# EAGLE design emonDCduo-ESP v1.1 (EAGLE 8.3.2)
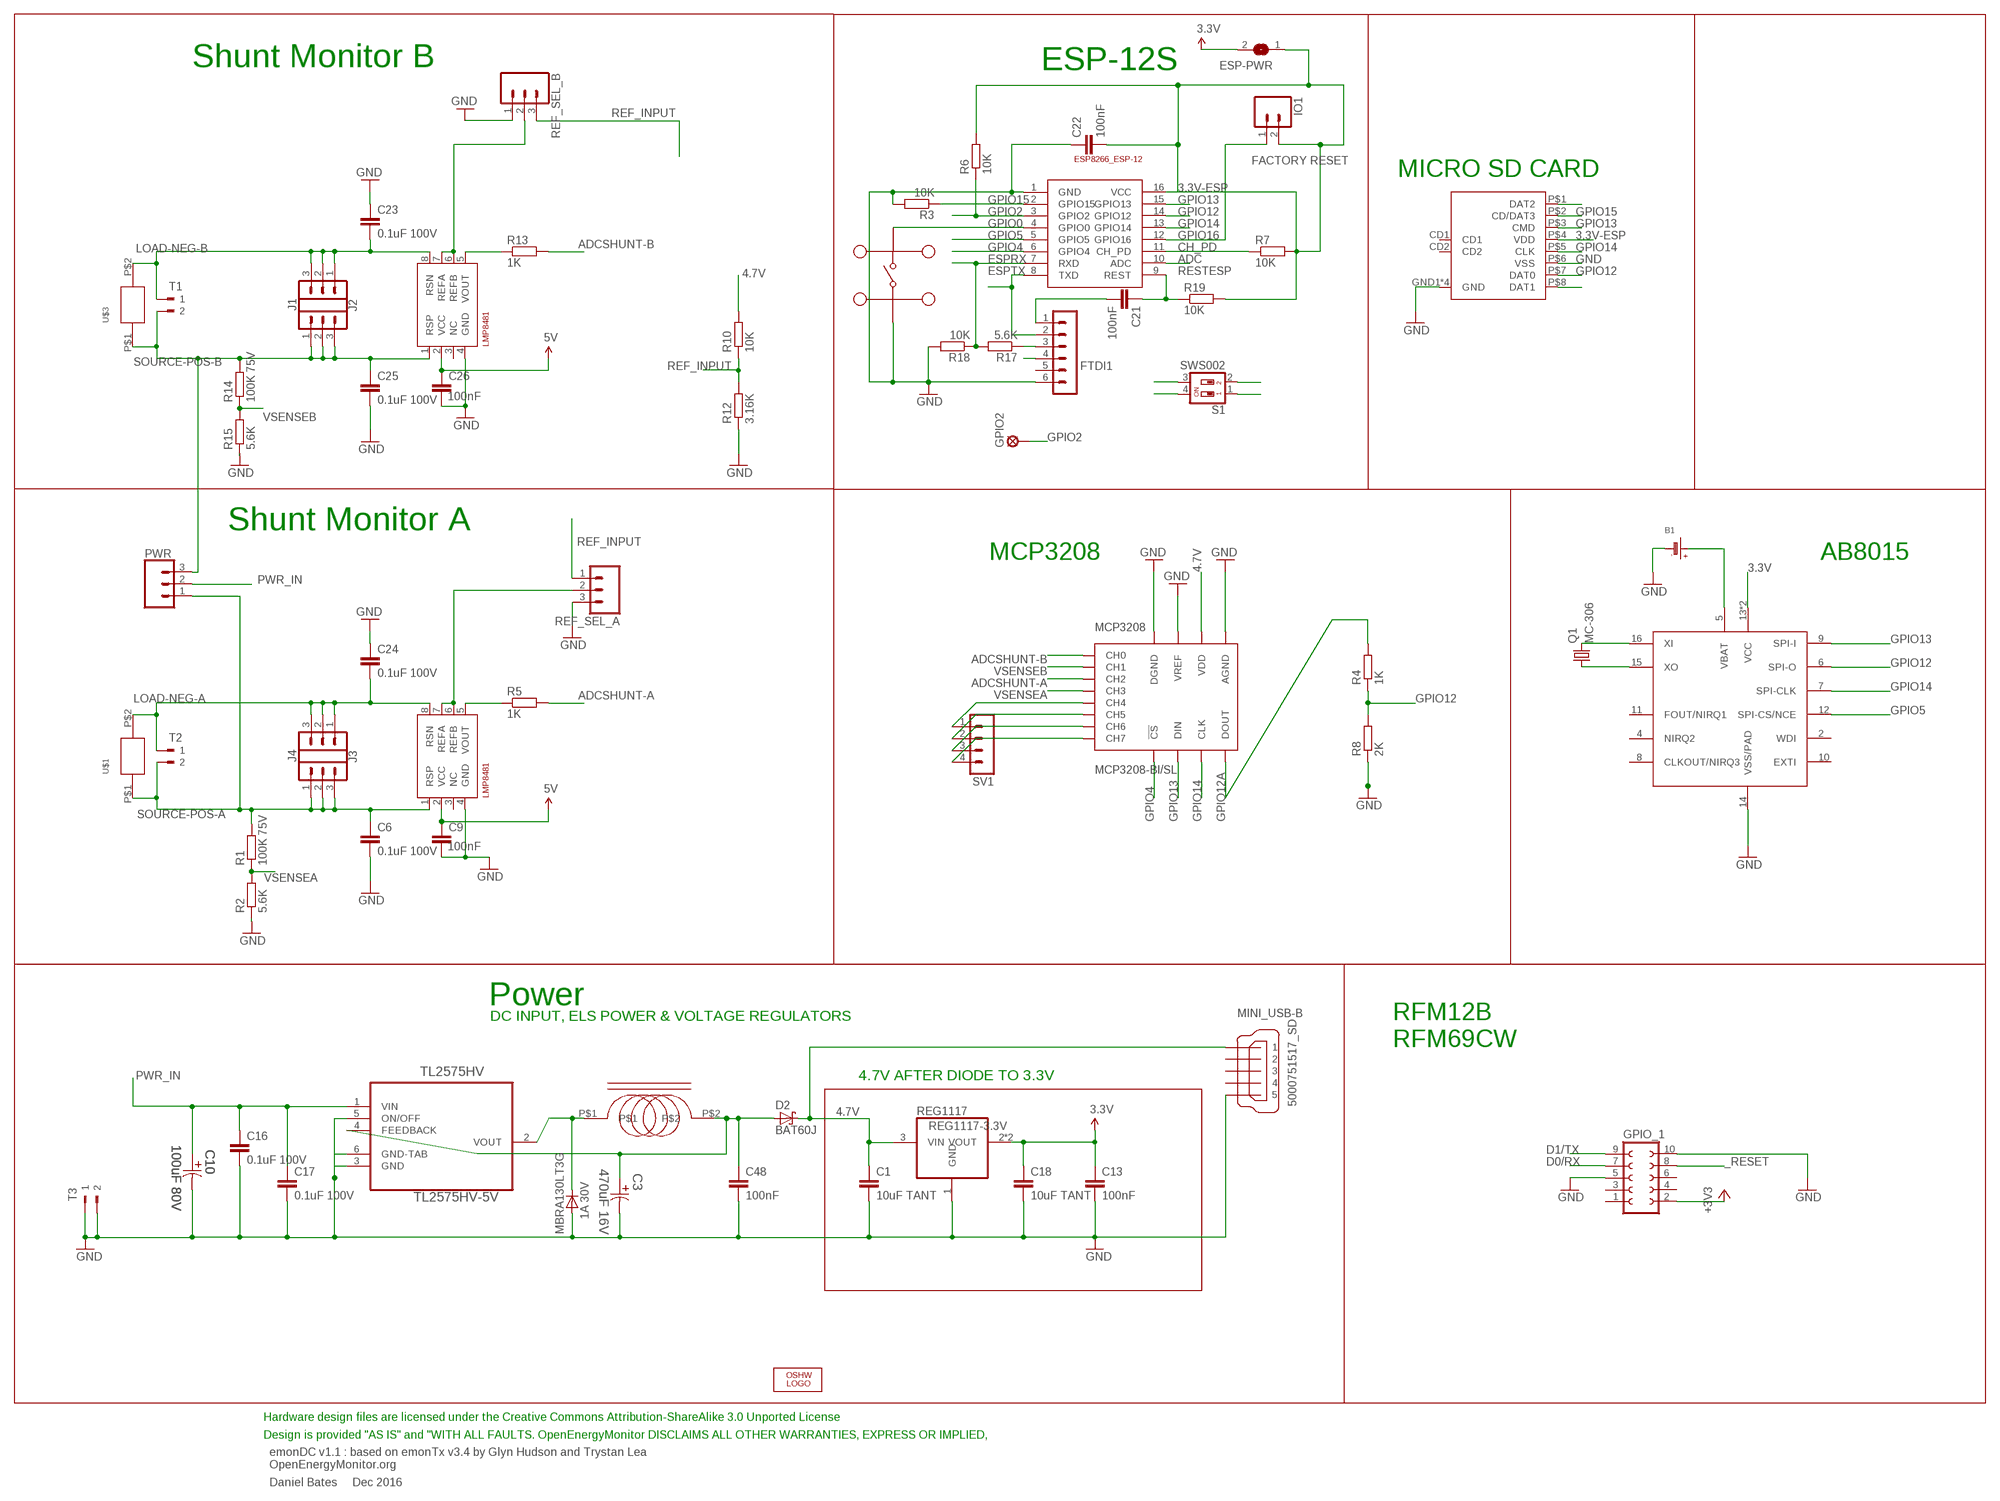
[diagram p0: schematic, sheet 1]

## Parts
AB8015  AB0815_RTC  [QFN16]
B1  BATTERYCR1220_SMT  [CR1220]
C1  10uF TANT  C-EUC0603  [C0603]
C3  470uF 16V  EEE-FK1C471P-CASE-F  [CAPAE830X1050N]
C6  0.1uF 100V  C-EUC0603  [C0603]
C9  100nF  C-EUC0603  [C0603]
C10  100uF 80V  EEV-FK1K101Q-CASE-H13  [CAPAE1350X1400N]
C13  100nF  C-EUC0603  [C0603]
C16  0.1uF 100V  C-EUC0603  [C0603]
C17  0.1uF 100V  C-EUC0603  [C0603]
C18  10uF TANT  C-EUC0603  [C0603]
C21  100nF  C-EUC0603  [C0603]
C22  100nF  C-EUC0603  [C0603]
C23  0.1uF 100V  C-EUC0603  [C0603]
C24  0.1uF 100V  C-EUC0603  [C0603]
C25  0.1uF 100V  C-EUC0603  [C0603]
C26  100nF  C-EUC0603  [C0603]
C48  100nF  C-EUC0603  [C0603]
D1  MBRA130LT3G  [DO-214]
D2  BAT60J  [SOD323_ST]
ESP-12  ESP8266_ESP-12  [ESP8266-ESP12]
ESP-PWR  SJ  [SJ]
FTDI1  FTDI-ESP  MA06-1  [MA06-1]
GPIO2  LSP11  [LSP11]
GPIO_1  FE05-2  [FE05-2]
I1  330uH  SRR0603-331KL  [SRR0603-331KL]
IO1  M02PTH  [1X02]
J1  CONN_03  [1X03]
J2  CONN_03  [1X03]
J3  CONN_03  [1X03]
J4  CONN_03  [1X03]
LOGO1  OSHW_LOGO_6MILX0200-NT  [OSHW_6X200_NOTEXT]
MC2  MC32882  [SWITCH_TACT_MULTICOMP]
MCP3208  MCP3208-BI/SL  [SOIC16]
MINI_USB-B  5000751517_SD  [5000751517_SD]
PWR  CONN_03  [1X03]
Q1  MC-306  [MC-306]
R1  100K 75V  R-EU_R0603  [R0603]
R2  5.6K  R-EU_R0603  [R0603]
R3  10K  R-EU_R0603  [R0603]
R4  1K  R-EU_R0603  [R0603]
R5  1K  R-EU_R0603  [R0603]
R6  10K  R-EU_R0603  [R0603]
R7  10K  R-EU_R0603  [R0603]
R8  2K  R-EU_R0603  [R0603]
R10  10K  R-EU_R0603  [R0603]
R12  3.16K  R-EU_R0603  [R0603]
R13  1K  R-EU_R0603  [R0603]
R14  100K 75V  R-EU_R0603  [R0603]
R15  5.6K  R-EU_R0603  [R0603]
R17  5.6K  R-EU_R0603  [R0603]
R18  10K  R-EU_R0603  [R0603]
R19  10K  R-EU_R0603  [R0603]
REF_SEL_A  2212S-02SG-85  CONN_03  [1X03]
REF_SEL_B  2212S-02SG-85  CONN_03  [1X03]
REG1117  REG1117-3.3V  REG1117-VOUT4  [SOT223]
S1  SWS002  [SMS-002]
SHUNTMON-A  LMP8481  LMP8481-H  [S-PDSO-G08]
SHUNTMON-B  LMP8481  LMP8481-H  [S-PDSO-G08]
SV1  MA04-1  [MA04-1]
T1  180-2  [180-2]
T2  180-2  [180-2]
T3  180-2  [180-2]
TL2575HV  TL2575HV-5V  TL2575HV-05IKTTR  [TO-263]
U$1  EBW_SERIES_10.5MM  [EBW_SERIES_10.5MM]
U$2  MOLEX_MICRO_SD_1040310811  [MOLEX_MICROSD_EXPOSED]
U$3  EBW_SERIES_10.5MM  [EBW_SERIES_10.5MM]

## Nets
3.3V: AB8015.13(VCC) AB8015.PAD(VCC) C13.1 C18.1 ESP-PWR.2 GPIO_1.2 REG1117.2(VOUT) REG1117.4(VOUT) ; supply symbol labelled +3V3
3.3V-ESP: C22.2 ESP-12.16(VCC) ESP-PWR.1 IO1.2 R6.2 R7.2 R19.2 U$2.P$4(VDD)
4.7V [power]: C1.1 C9.1 C26.1 D2.C FTDI1.4 MCP3208.16(VDD) MINI_USB-B.VBUS R10.2 REG1117.3(VIN) SHUNTMON-A.2(VCC) SHUNTMON-B.2(VCC) ; supply symbol labelled 5V
5.0V [power]: C3.1 C48.1 D2.A I1.P$2 TL2575HV.4(FEEDBACK)
_RESET: GPIO_1.8
ADC: ESP-12.10(ADC)
ADCSHUNT-A: MCP3208.3(CH2) R5.2
ADCSHUNT-B: MCP3208.1(CH0) R13.2
CH_PD: ESP-12.11(CH_PD) R7.1
D0/RX: GPIO_1.7 S1.2
D1/TX: GPIO_1.9 S1.1
ESPRX: ESP-12.7(RXD) R17.2 R18.1 S1.4
ESPTX: ESP-12.8(TXD) FTDI1.2 S1.3
GND [thin_power]: AB8015.14(VSS/PAD) B1.- C1.2 C3.2 C6.2 C9.2 C10.2 C13.2 C16.2 C17.2 C18.2 C22.1 C23.1 C24.1 C25.2 C26.2 C48.2 D1.P$2(A) ESP-12.1(GND) FTDI1.6 GPIO_1.5 GPIO_1.10 MC2.P$1 MC2.P$2 MCP3208.9(DGND) MCP3208.14(AGND) MCP3208.15(VREF) MINI_USB-B.GND1 MINI_USB-B.GND2 MINI_USB-B.GND3 R2.1 R3.2 R8.1 R12.1 R15.1 R18.2 REF_SEL_A.3 REF_SEL_B.1 REG1117.1(GND) SHUNTMON-A.4(GND) SHUNTMON-B.4(GND) T3.1 T3.2 TL2575HV.3(GND) TL2575HV.5(ON/OFF) TL2575HV.6(GND-TAB) U$2.GND1(GND) U$2.GND2(GND) U$2.GND3(GND) U$2.GND4(GND) U$2.P$6(VSS)
GPIO0: ESP-12.4(GPIO0) MC2.P$3 MC2.P$4
GPIO2: ESP-12.3(GPIO2) GPIO2.MP R6.1
GPIO4: ESP-12.6(GPIO4) MCP3208.10(!CS)
GPIO5: AB8015.12(SPI-CS/NCE) ESP-12.5(GPIO5)
GPIO12: AB8015.6(SPI-O) ESP-12.14(GPIO12) R4.1 R8.2 U$2.P$7(DAT0)
GPIO12A: MCP3208.12(DOUT) R4.2
GPIO13: AB8015.9(SPI-I) ESP-12.15(GPIO13) MCP3208.11(DIN) U$2.P$3(CMD)
GPIO14: AB8015.7(SPI-CLK) ESP-12.13(GPIO14) MCP3208.13(CLK) U$2.P$5(CLK)
GPIO15 [thin_power]: ESP-12.2(GPIO15) R3.1 U$2.P$2(CD/DAT3)
GPIO16: ESP-12.12(GPIO16) IO1.1
IND: D1.P$1(C) I1.P$1 TL2575HV.2(VOUT)
LOAD-NEG-A: C24.2 J4.1 J4.2 J4.3 SHUNTMON-B.8(RSN) T2.1 U$1.P$2
LOAD-NEG-B: C23.2 J1.1 J1.2 J1.3 SHUNTMON-A.8(RSN) T1.1 U$3.P$2
N$1: MCP3208.5(CH4) SV1.1
N$3: MCP3208.6(CH5) SV1.2
N$4: R13.1 SHUNTMON-A.5(VOUT)
N$5: MCP3208.7(CH6) SV1.3
N$6: R5.1 SHUNTMON-B.5(VOUT)
N$7: U$2.P$1(DAT2)
N$9: MCP3208.8(CH7) SV1.4
N$20: AB8015.5(VBAT) B1.+$1(+)
N$22: AB8015.16(XI) Q1.4
N$23: AB8015.15(XO) Q1.1
N$30: C21.2 FTDI1.1
N$32: U$2.P$8(DAT1)
N$36: FTDI1.3 R17.1
PWR_IN: C10.1 C16.1 C17.1 PWR.2 TL2575HV.1(VIN)
REF_A_INPUT [thin_power]: REF_SEL_A.2 SHUNTMON-B.6(REFB) SHUNTMON-B.7(REFA)
REF_B_INPUT: REF_SEL_B.2 SHUNTMON-A.6(REFB) SHUNTMON-A.7(REFA)
REF_INPUT: R10.1 R12.2 REF_SEL_A.1 REF_SEL_B.3
RESTESP: C21.1 ESP-12.9(REST) R19.1
SOURCE-POS-A: C6.1 J3.1 J3.2 J3.3 PWR.1 R1.2 SHUNTMON-B.1(RSP) T2.2 U$1.P$1
SOURCE-POS-B: C25.1 J2.1 J2.2 J2.3 PWR.3 R14.2 SHUNTMON-A.1(RSP) T1.2 U$3.P$1
VSENSEA: MCP3208.4(CH3) R1.1 R2.2
VSENSEB: MCP3208.2(CH1) R14.1 R15.2
Unconnected: AB8015.2(WDI) AB8015.4(NIRQ2) AB8015.8(CLKOUT/NIRQ3) AB8015.10(EXTI) AB8015.11(FOUT/NIRQ1) FTDI1.5 GPIO_1.1 GPIO_1.3 GPIO_1.4 GPIO_1.6 MINI_USB-B.D+ MINI_USB-B.D- MINI_USB-B.ID SHUNTMON-A.3(NC) SHUNTMON-B.3(NC) U$2.CD1 U$2.CD2

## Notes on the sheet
- Shunt Monitor B | ESP-12S
- FACTORY RESET
- MICRO SD CARD
- Shunt Monitor A
- MCP3208 | AB8015
- Power
- DC INPUT, ELS POWER & VOLTAGE REGULATORS
- RFM12B
  RFM69CW
- 4.7V AFTER DIODE TO 3.3V
- Hardware design files are licensed under the Creative Commons Attribution-ShareAlike 3.0 Unported License
- Design is provided "AS IS" and "WITH ALL FAULTS. OpenEnergyMonitor DISCLAIMS ALL OTHER WARRANTIES, EXPRESS OR IMPLIED,
- emonDC v1.1 : based on emonTx v3.4 by Glyn Hudson and Trystan Lea
  OpenEnergyMonitor.org
- Daniel Bates     Dec 2016

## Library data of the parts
AB8015 = AB0815 RTC:AB0815_RTC
B1 = microbuilder:BATTERY: CR1220 SMT - Digikey: 3001K-ND
C1 C13 C16-C18 C21 C22 C48 = rcl:C-EU: CAPACITOR, European symbol
C3 = Panasonic-EEEFK_EEEFP:EEE-: Aluminum Electrolytic Capacitors,Surface Mount Type; MPN: EEE-FK1C471P; OC_FARNELL: 9695710; OC_NEWARK: 96K9385; PACKAGE: CASE-F; SUPPLIER: PANASONIC; TOLERANCE: ±20 %; VALUE: 470UF; VOLTAGERATING: 16V
C6 C9 C23-C26 = rcl:C-EU: CAPACITOR, European symbol; MPN: C1608X7S2A104K080AB
C10 = Panasonic-EEE-EEV-EEF-ECQ:EEV-: Aluminum Electrolytic Capacitors,Surface Mount Type; MPN: EEVFK1K101Q; OC_FARNELL: 9696113; OC_NEWARK: 96K9484; SUPPLIER: PANASONIC; TOLERANCE: ±20 %; VALUE: 100UF; VOLTAGERATING: 80V
D1 = CASE 403D Diode:MBRA130LT3G: Fast switching diode; MF: ON SEMICONDUCTOR; MPN: MBRA130LT3G; OC_FARNELL: 9555978
D2 = diode:BAT60J: Schottky barrier diode
ESP-12 = ESP8266-ESP12:ESP8266_ESP-12
ESP-PWR = jumper:SJ: SMD solder JUMPER
FTDI1 = JeeLabs:MA06-1: PIN HEADER
GPIO2 = solpad:LSP11: SOLDER PAD
GPIO_1 = con-lsta:FE05-2: FEMALE HEADER; OC_FARNELL: unknown; OC_NEWARK: unknown
I1 = SRR0603-331KL:SRR0603-331KL: SRR0603-331KL; INDUCTANCE: 330uH; MF: BOURNS; MPN: SRR0603-331KL; OC_FARNELL: 2333890
IO1 = SparkFun:M02: Header 2
J1-J4 PWR = SparkFun-Connectors:CONN_03: Multi connection point. Often used as Generic Header-pin footprint for 0.1 inch spaced/style header connections On any of the 0.1 inch spaced packages, you can populate with these: Break Away Headers - Straight (PRT-00116) Break Away Male Headers - Right Angle (PRT-00553) Female Headers (PRT-00115)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
LOGO1 = ohw-logo:OSHW_LOGO_6MIL; OC_FARNELL: unknown
MC2 = multicomp tact switch:MC32882
MCP3208 = MCP3208:MCP3208
MINI_USB-B = 5000751517_sd:5000751517_SD
Q1 = crystal:MC-306: kHz RANGE CRYSTAL UNIT SMD; MPN: MC-306 60.0KHZ 100PPM ,12.5PF; OC_FARNELL: 1278040; OC_NEWARK: 31M5576
R1 R14 = rcl:R-EU_: RESISTOR, European symbol; MPN: MCWR06X1003FTL
R2 R4 R8 R15 = rcl:R-EU_: RESISTOR, European symbol; MPN: MCWR06X5901FTL
R3 R5-R7 R10 R12 R13 R17-R19 = rcl:R-EU_: RESISTOR, European symbol
REF_SEL_A REF_SEL_B = SparkFun-Connectors:CONN_03: Multi connection point. Often used as Generic Header-pin footprint for 0.1 inch spaced/style header connections On any of the 0.1 inch spaced packages, you can populate with these: Break Away Headers - Straight (PRT-00116) Break Away Male Headers - Right Angle (PRT-00553) Female Headers (PRT-00115)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; MF: MULTICOMP; MPN: 2212S-02SG-85; OC_FARNELL: 1593458
REG1117 = burr-brown:REG1117-VOUT4: 800mA and 1A Low Dropout (LDO) Positive Regulator 1.8V, 2.5V, 2.85V, 3.3V, 5V, and Adj; MF: TEXAS INSTRUMENTS; MPN: REG1117; OC_FARNELL: 1097566; OC_NEWARK: 14P6981
S1 = smd-special:SWS002: SMD Dip Switch 2 pol.
SHUNTMON-A = lmp8481b:LMP8481: LMP8481MM-H/NOPB 100V/V; MF: TEXAS INSTRUMENTS; MPN: LMP8481MME-S/NOPB; OC_FARNELL: 2322044
SHUNTMON-B = lmp8481b:LMP8481: LMP8481MM-H/NOPB 100V/V; MF: TEXAS INSTRUMENTS; MPN: LMP8481MME-H/NOPB; OC_FARNELL: 2322044
SV1 = con-lstb:MA04-1: PIN HEADER; OC_FARNELL: unknown; OC_NEWARK: unknown
T1-T3 = con-weidmueller-sl35:180-2: WEIDMUELLER CLAMP CONNECTOR; OC_FARNELL: unknown; OC_NEWARK: unknown
TL2575HV = TL2575HV:TL2575HV; MF: TEXAS INSTRUMENTS; MPN: LM2575HVS-15/NOPB; OC_FARNELL: 2492609
U$1 U$3 = EBW series shunt:EBW_SERIES_10.5MM
U$2 = MOLEX MICRO SD [exposed pins]:MOLEX_MICRO_SD_1040310811

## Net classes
2 thin_power: width 0.254 mm

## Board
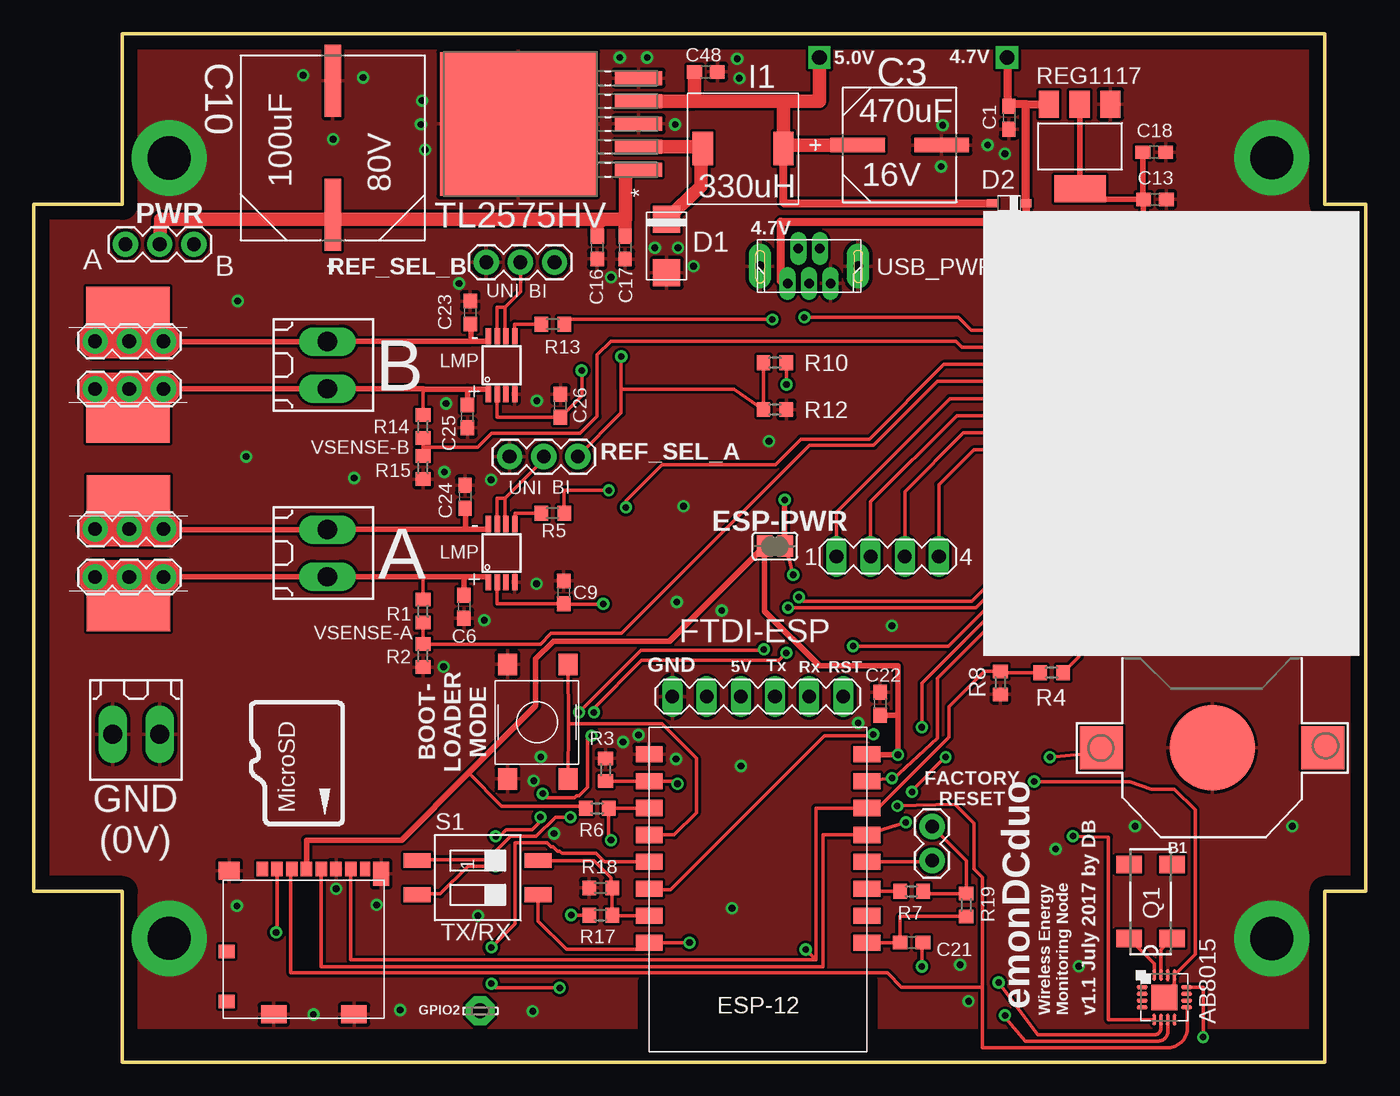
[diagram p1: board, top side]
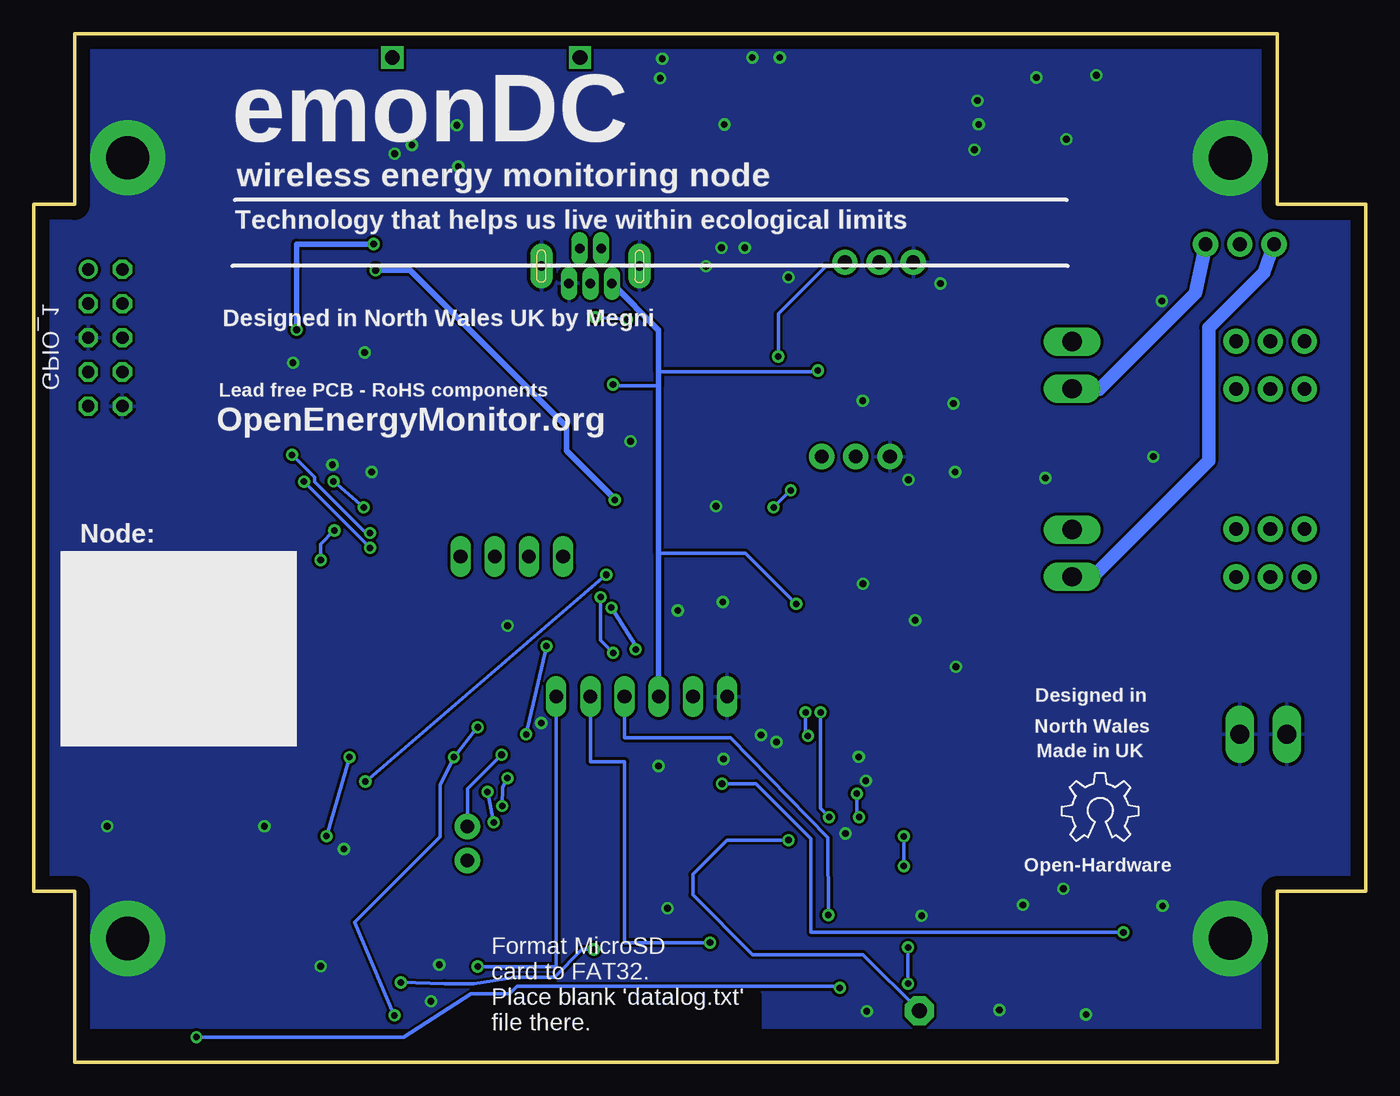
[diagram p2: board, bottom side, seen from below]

Size 99.06 x 76.45 mm. Coordinates in mm from the lower left corner, seen from the top.
Outline: 6.6,63.75 6.6,76.45 96.01,76.45 96.01,63.75 99.06,63.75 99.06,12.7 96.01,12.7 96.01,0 6.6,0 6.6,12.7 0,12.7 0,63.75 6.6,63.75
Copper layers (1*16): Top 0.035mm / dielectric 1.5mm / Bottom 0.035mm
Design rules "default *": minimum track width 10mil, minimum drill 19mil, track to track 8mil, track to pad 8mil, pad to pad 8mil, via to via 8mil, smd to smd 8mil, copper to edge 40mil, drill to drill 8mil, minimum pad ring 10mil, minimum via ring 8mil, stop-mask expansion 4mil, vias tented up to drill 0mil, thermal gap 10mil
tRestrict: area 45.2,2.3 to 62.5,6.1
bRestrict: area 45.2,2.3 to 62.5,5.1

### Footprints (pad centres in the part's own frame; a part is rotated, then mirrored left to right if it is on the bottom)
QFN16 = smd 0.85 x 0.3: 1 -1.655,0.75; 2 -1.655,0.25; 3 -1.655,-0.25; 4 -1.655,-0.75; 9 1.655,-0.75; 10 1.655,-0.25; 11 1.655,0.25; 12 1.655,0.75 | smd 0.3 x 0.85: 5 -0.75,-1.655; 6 -0.25,-1.655; 7 0.25,-1.655; 8 0.75,-1.655; 13 0.75,1.655; 14 0.25,1.655; 15 -0.25,1.655; 16 -0.75,1.655 | smd 1.9 x 1.9: PAD 0,0
CR1220 = smd 3.2 x 3.2: +$1 -8.225,0; +$2 8.225,0 | smd 6.35 x 6.35: - 0,0
C0603 = smd 1.1 x 1: 1 -0.85,0; 2 0.85,0
CAPAE830X1050N = smd 4.064 x 1.092: 1 -3.124,0; 2 3.124,0
CAPAE1350X1400N = smd 5.359 x 1.194: 1 -4.978,0; 2 4.978,0
DO-214 = smd 2 x 2: P$1 -2,0; P$2 2,0
SOD323_ST = smd 0.8 x 0.6: A 1.25,0; C -1.25,0
ESP8266-ESP12 = smd 2 x 1.2: 1 16.2,2; 2 16.2,4; 3 16.2,6; 4 16.2,8; 5 16.2,10; 6 16.2,12; 7 16.2,14; 8 16.2,16; 9 0,16; 10 0,14; 11 0,12; 12 0,10; 13 0,8; 14 0,6; 15 0,4; 16 0,2
SJ = smd 1.168 x 1.6: 1 -0.762,0; 2 0.762,0
MA06-1 = drill 1.016 long: 1 0,0; 2 2.54,0; 3 5.08,0; 4 7.62,0; 5 10.16,0; 6 12.7,0
LSP11 = drill 1.118 pad 2.159 octagon: MP 0,0
FE05-2 = drill 0.914: 1 -5.08,1.27 | drill 0.914 octagon: 2 -5.08,-1.27; 3 -2.54,1.27; 4 -2.54,-1.27; 5 0,1.27; 6 0,-1.27; 7 2.54,1.27; 8 2.54,-1.27; 9 5.08,1.27; 10 5.08,-1.27
SRR0603-331KL = smd 1.5 x 2.5: P$1 -3,0; P$2 3,0
1X02 = drill 1.016 pad 1.88: 1 0,0; 2 2.54,0
1X03 = drill 1.016 pad 1.88: 1 0,0; 2 2.54,0; 3 5.08,0
SWITCH_TACT_MULTICOMP = smd 1.6 x 1.4: P$1 -1.1,5.3; P$2 7.4,5.3; P$3 -1.1,0.8; P$4 7.4,0.8
SOIC16 = smd 0.635 x 1.524: 1 -4.445,-2.695; 2 -3.175,-2.695; 3 -1.905,-2.695; 4 -0.635,-2.695; 5 0.635,-2.695; 6 1.905,-2.695; 7 3.175,-2.695; 8 4.445,-2.695; 9 4.445,2.695; 10 3.175,2.695; 11 1.905,2.695; 12 0.635,2.695; 13 -0.635,2.695; 14 -1.905,2.695; 15 -3.175,2.695; 16 -4.445,2.695
5000751517_SD = drill 0.7 pad 1.016 long: D+ 0,-1.3; D- -0.8,1.3; GND1 1.6,-1.3; ID 0.8,1.3; VBUS -1.6,-1.3 | drill 0.7 pad 1.676 long: GND2 3.65,0; GND3 -3.65,0
MC-306 = smd 1.3 x 1.9: 1 -2.75,-1.6; 2 2.75,-1.6; 3 2.75,1.6; 4 -2.75,1.6
R0603 = smd 1 x 1.1: 1 -0.85,0; 2 0.85,0
SOT223 = smd 1.499 x 2.007: 1 -2.261,-3.15; 2 0.025,-3.15; 3 2.311,-3.15 | smd 3.81 x 2.007: 4 0,3.15
SMS-002 = smd 1.092 x 2.007: 1 -1.27,-4.496; 2 1.27,-4.496; 3 1.27,4.496; 4 -1.27,4.496
S-PDSO-G08 = smd 0.4 x 1.2: 1 -0.975,-2.157; 2 -0.325,-2.157; 3 0.325,-2.157; 4 0.975,-2.157; 5 0.975,2.157; 6 0.325,2.157; 7 -0.325,2.157; 8 -0.975,2.157
MA04-1 = drill 1.016 long: 1 -3.81,0; 2 -1.27,0; 3 1.27,0; 4 3.81,0
180-2 = drill 1.422 long: 1 -1.75,0; 2 1.75,0
TO-263 = smd 1.041 x 3.505: 1 -3.404,-8.788; 2 -1.702,-8.788; 3 0,-8.788; 4 1.702,-8.788; 5 3.404,-8.788 | smd 10.668 x 11.659: 6 0,0.152
EBW_SERIES_10.5MM = smd 3 x 6.2: P$1 -4.3,0; P$2 4.3,0
MOLEX_MICROSD_EXPOSED = smd 1.195 x 1.005: CD1 5.349,0.435; CD2 5.349,4.135 | smd 1.907 x 1.348: GND1 -4.112,5.104; GND2 1.853,5.104 | smd 1.17 x 1.793: GND3 -6.134,-5.352 | smd 1.551 x 1.348: GND4 5.167,-5.577 | smd 0.851 x 1.092: P$1 2.707,-5.703; P$2 1.617,-5.703; P$3 0.522,-5.699; P$4 -0.586,-5.701; P$5 -1.676,-5.703; P$6 -2.769,-5.703; P$7 -3.875,-5.701 | smd 0.749 x 1.092: P$8 -4.935,-5.701

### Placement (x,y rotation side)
AB8015  84.07,4.83 0 top
B1  87.63,23.37 0 top
C1  72.52,70.21 270 top
C3  64.39,68.17 0 top
C6  32,33.86 270 top
C9  39.42,34.93 90 top
C10  22.25,67.96 90 top
C13  83.38,64.13 0 top
C16  41.9,60.55 270 top
C17  43.97,60.55 270 top
C18  83.32,67.64 0 top
C21  65.28,8.89 0 top
C22  62.94,26.64 270 top
C23  32.46,55.73 270 top
C24  32.08,42.04 270 top
C25  32.26,48.01 270 top
C26  39.17,48.8 90 top
C48  49.99,73.61 0 top
D1  47.06,60.67 270 top
D2  72.53,63.85 180 top
ESP-12  61.98,24.89 180 top
ESP-PWR  55.12,38.35 0 top
FTDI1  60.2,27.18 180 top
GPIO2  33.21,3.81 0 top
GPIO_1  93.73,53.85 270 top
I1  52.76,67.91 0 top
IO1  66.8,14.99 90 top
J1  4.57,53.59 0 top
J2  4.57,50.04 0 top
J3  4.57,36.07 0 top
J4  4.57,39.62 0 top
LOGO1  22.6,16.43 0 bottom
MC2  40.53,22.17 90 top
MCP3208  74.54,49.96 270 top
MINI_USB-B  57.66,59.18 0 top
PWR  6.84,60.8 0 top
Q1  83.06,11.94 90 top
R1  28.96,33.53 90 top
R2  28.96,30.23 90 top
R3  42.53,21.74 90 top
R4  75.69,28.96 0 top
R5  38.6,40.81 0 top
R6  41.91,18.87 180 top
R7  65.28,12.7 0 top
R8  71.88,28.19 90 top
R10  55.12,52 0 top
R12  55.12,48.51 180 top
R13  38.61,54.86 0 top
R14  28.96,47.24 90 top
R15  28.96,44.2 90 top
R17  42.16,10.92 0 top
R18  42.16,12.95 180 top
R19  69.34,11.68 90 top
REF_SEL_A  40.47,45.01 180 top
REF_SEL_B  33.65,59.46 0 top
REG1117  77.8,68.07 180 top
S1  33.02,13.72 270 top
SHUNTMON-A  34.8,51.82 0 top
SHUNTMON-B  34.8,37.85 0 top
SV1  63.5,37.59 0 top
T1  21.84,51.82 270 top
T2  21.84,37.85 270 top
T3  7.62,24.38 180 top
TL2575HV  36.19,69.74 90 top
U$1  7.05,37.82 90 top
U$2  19.71,8.66 180 top
U$3  7.02,51.83 90 top

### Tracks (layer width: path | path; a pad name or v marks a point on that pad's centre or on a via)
3.3V  (via drill 0.5)
  Top 0.254: AB8015.13 84.84,5.84 84.52,5.53 84.52,4.89 84.2,4.89 AB8015.PAD | 55.94,38.39 ESP-PWR.2 55.94,38.23 56.45,36.29 | 92.46,58.86 GPIO_1.2 | v74.39,20.86 81.5,20.86 83.09,20.29 84.84,20.29 86.36,18.76 86.36,8.02 AB8015.13 | 56.52,36.32 56.61,36.23 | 84.84,6.64 AB8015.13
  Top 0.406: REG1117.2 77.76,71.22 | 82.51,58.86 92.46,58.86 | 82.51,58.86 v73.63,58.86 | REG1117.4 78.6,64.13 C13.1 | C13.1 82.47,64.18 C18.1 | C13.1 82.51,64.11 82.51,58.86 | v55.84,41.8 55.84,38.49 55.94,38.39 | 56.45,36.29 56.48,36.26 v56.48,36.23 56.48,36.29 56.52,36.32
  Bottom 0.254: v56.48,36.23 v74.39,20.86
  Bottom 0.406: v73.63,58.86 71.06,58.86 59.44,47.24 59.44,45.45 55.87,41.89 55.87,41.83 v55.84,41.8
3.3V-ESP  (via drill 0.5)
  Top 0.254: R7.2 66.13,12.53 R19.2 69.34,14.99 IO1.2 | R6.2 40.89,19.04 34.81,19.04 32.35,21.5
  Top 0.406: 64.26,25.91 64.26,29.46 58.42,29.46 54.36,33.53 ESP-PWR.1 47.29,31.28 38.65,31.28 37.34,29.97 37.34,26.49 32.35,21.5 27.35,16.51 20.3,16.51 U$2.P$4 | 64.26,25.91 v64.26,22.86 62.01,22.86 ESP-12.16 | C22.2 64.15,25.8 64.26,25.91
  Bottom 0.254: v64.26,22.86 66.8,20.32 IO1.2
4.7V  (via drill 0.5, 1.1)
  Top 0.254: SHUNTMON-A.2 34.47,47.95 C26.1 40.76,49.54 40.76,51.36 40.75,51.36 v40.75,51.41 | SHUNTMON-B.2 34.47,34.08 C9.1 39.46,34.04 42.42,34.04 42.39,34.07 v42.36,34.07 | R10.2 55.98,51.98 v55.98,50.38
  Top 0.406: D2.C 73.96,63.85 | 72.39,71.06 C1.1 72.52,71.22 | 73.78,62.48 73.79,62.48 v73.79,60.81 | v79.5,54.44 77.27,54.44 MCP3208.16 | MINI_USB-B.VBUS 55.86,58.08 55.56,58.08
  Top 0.61: v72.39,74.68 72.39,71.06 | 73.78,71.22 D2.C 73.78,62.48 55.56,62.48 55.56,58.08 | 73.78,71.22 REG1117.3 | 73.78,71.22 72.52,71.22
  Bottom 0.254: v55.98,50.38 55.9,50.29 52.58,50.29 | v40.75,51.41 40.85,51.31 52.58,51.31 | v42.36,34.07 46.14,37.85 52.58,37.85
  Bottom 0.406: v79.5,54.44 79.5,60.81 v73.79,60.81 | FTDI1.4 52.58,37.85 52.58,50.29 52.58,51.31 52.58,54.4 MINI_USB-B.VBUS
5.0V  (via drill 1.1)
  Top 0.61: D2.A 55.76,63.85 I1.P$2
  Top 1.016: TL2575HV.4 49.14,71.44 | 49.14,71.44 C48.1 | 55.76,71.44 I1.P$2 55.5,68.17 C3.1 | 55.76,71.44 49.14,71.44 | v58.42,74.68 58.42,71.44 55.76,71.44
ADCSHUNT-A  (via drill 0.48)
  Top 0.254: v42.77,42.51 39.43,42.51 39.43,40.93 R5.2 | v44.04,41.24 44.04,41.72 46.74,44.42 55.15,44.42 57.05,46.32 62.14,46.32 67.69,51.88 71.82,51.88 MCP3208.3
  Bottom 0.254: v44.04,41.24 v42.77,42.51
ADCSHUNT-B  (via drill 0.48)
  Top 0.254: v57.31,55.37 68.77,55.37 69.72,54.42 71.82,54.42 MCP3208.1 | R13.2 39.43,54.9 39.43,55.21 54.99,55.21 v54.92,55.21
  Bottom 0.254: v54.92,55.21 v57.31,55.37
CH_PD
  Top 0.254: ESP-12.11 61.98,12.7 R7.1
D0/RX  (via drill 0.48)
  Top 0.254: v34.35,14.57 32.29,14.57 30.23,12.51 28.64,12.51 S1.2 | v34.35,16.8 34.67,16.8 35.15,17.27 37.05,17.27 37.69,17.91 v37.69,18.23 | v37.85,19.97 38.16,19.65 40.23,19.65 40.39,19.81 40.55,19.81 41.18,20.45 41.18,24.26 v41.5,24.26 | v41.66,26 41.66,26.32 45.21,29.88 55.42,29.88 v55.97,30.43 55.96,30.22 | v56.9,34.58 57.21,34.26 69.75,34.26 73.25,37.75 73.25,39.34 v74.04,39.34 | v79.85,45.15 79.66,44.89 82.52,47.75 89.92,47.75 92.2,50.04 93.22,50.04 94.23,51.05 94.8,51.05 95,51.25 GPIO_1.7
  Bottom 0.254: v34.35,16.8 v34.35,14.57 | v37.69,18.23 37.85,18.38 v37.85,19.97 | v41.5,24.26 41.66,24.42 v41.66,26 | v74.04,39.34 74.36,39.34 78.17,43.15 78.17,43.47 v79.85,45.15 | v55.97,30.43 56.9,31.35 v56.9,34.58
D1/TX  (via drill 0.48)
  Top 0.254: v39.91,18.23 38.8,18.23 37.37,16.8 35.47,16.8 33.72,15.05 28.64,15.05 S1.1 | v40.55,26 45.15,30.61 54.22,30.61 v54.29,30.68 | v56.1,33.78 70.07,33.78 74.04,37.75 v74.04,38.23 | v78.96,43.15 82.3,46.48 93.98,46.48 95,47.5 GPIO_1.9 95,48.7
  Bottom 0.254: v39.91,18.23 40.55,18.86 v40.55,26 | v54.29,30.68 54.32,31.02 v56.1,33.78 | v78.96,43.15 v74.04,38.23
ESPRX
  Top 0.254: ESP-12.7 42.79,10.89 R17.2 R18.1 42.93,13.04 42.93,13.72 41.66,14.99 S1.4
ESPTX  (via drill 0.5)
  Top 0.254: v48.77,8.89 ESP-12.8 45.27,8.38 39.62,8.38 37.52,10.49 S1.3
  Bottom 0.254: v48.77,8.89 55.12,8.89 55.12,22.35 57.66,22.35 FTDI1.2
GND  (via drill 0.5, 3.2 pad 5.59)
  Top 0.254: ESP-12.1 46.06,22.61
  Top 0.406: U$2.GND2 | U$2.P$6 22.48,14.39 | 25.86,13.97 25.91,13.97 25.96,14.02
  other vias: 10.08,67.21 92.07,67.23 52.47,73.15 10.08,9.2 92.07,9.2 33.51,32.85 15.17,56.58 30.55,43.87 37.41,49.17 70.94,68.18 30.66,48.96 37.39,35.57 47.77,22.53 51.93,11.44 22.49,12.89 42.93,58.34 49.07,59.16 67.59,69.65 47.7,69.7 28.88,71.47 20.04,73.36 24.49,73.2 15.81,45.01 30.48,29.4 34.01,43.3 20.81,3.54 47.92,60.54 44.98,24.32 25.51,11.7 61.31,25.22 15.12,11.62 38.69,17 31.64,57.88 23.83,43.43 43.83,23.8 37.18,20.93 37.71,22.7 33.04,10.88 27.25,3.88 37.11,3.79 46.19,60.53 67.48,66.58 72.22,67.52 52.32,74.58 29.11,67.83 28.79,69.71 43.59,74.69 45.62,74.69 22.27,68.6 68.89,7.24 77.71,7.13 75.99,15.85 93.58,17.54 81.9,17.54 48.33,41.33 47.82,34.21 51.17,33.58 63.82,32.44 69.52,4.54 52.6,22.02 73.93,43.87 79.77,52 74.44,52.76 76.85,44.42 54.68,46.15
  pour Bottom (isolate 0.127): 6.86,76.2 6.86,63.5 0.25,63.5 0.25,12.95 6.86,12.95 6.86,2.54 95.76,2.54 95.76,12.95 98.81,12.95 98.81,63.5 95.76,63.5 95.76,76.2
  pour Top (isolate 0.127): 6.86,76.2 6.86,63.5 0.25,63.5 0.25,12.95 6.86,12.95 6.86,2.54 95.76,2.54 95.76,12.95 98.81,12.95 98.81,63.5 95.76,63.5 95.76,76.2
GPIO0
  Top 0.254: MC2.P$3 39.77,25.15 | 39.77,25.15 MC2.P$4 | ESP-12.4 47.63,16.89 49.28,18.54 49.28,22.61 46.74,25.15 39.77,25.15
GPIO2  (via drill 0.5)
  Top 0.254: ESP-12.3 42.78,18.89 R6.1 42.76,16.68 v42.93,16.51
  Bottom 0.254: v42.93,16.51 47.5,16.51 50.04,13.97 50.04,12.45 45.6,8.01 37.4,8.01 GPIO2.MP
GPIO4  (via drill 0.48)
  Top 0.254: 45.32,12.89 ESP-12.6 45.78,12.83 47.37,12.83 58.8,24.26 62.14,24.26 v62.44,24.38 | v74.52,41.24 74.83,40.93 74.83,37.75 68.01,30.93 v60.93,30.93 | MCP3208.10 77.38,46.64 77.69,46.64 78.33,46.01 78.33,45 77.66,44.33 77.66,43.91 76.92,43.17 v76.76,43.17
  Bottom 0.254: v74.52,41.24 v76.76,43.17 | v62.44,24.38 v60.93,30.93
GPIO5  (via drill 0.48)
  Top 0.254: v86.95,1.87 86.96,2.76 86.96,5.58 AB8015.12 | v34.04,8.54 35.78,10.29 35.78,16.32 38.16,16.32 38.48,16 38.64,16 38.96,15.68 39.12,15.68 39.28,15.53 41.82,15.53 42.45,14.89 45.62,14.89 ESP-12.5 | v34.04,5.84 34.35,5.53 v39.12,5.53
  Bottom 0.254: v34.04,8.54 v34.04,5.84 | v86.95,1.87 85.63,1.87 71.53,1.87 66.55,5.08 63.68,5.08 63.13,5.63 39.22,5.63 v39.12,5.53
GPIO12  (via drill 0.5)
  Top 0.254: 58.17,7.62 23.59,7.62 U$2.P$7 | 58.17,7.62 58.17,18.89 ESP-12.14 61.98,18.86 62.77,18.86 68.07,24.16 68.07,26.42 70.7,29.04 R8.2 71.97,28.96 R4.1 | AB8015.6 83.82,2.54 arc-90 83.31,2.03 74.68,2.03 v71.75,5.93 | 58.17,7.62 v57.4,8.38
  Bottom 0.254: v71.75,5.93 68.52,5.84 67.24,5.83 66.3,5.83 63.27,6.33 60.34,6.33 58.28,8.38 v57.4,8.38
GPIO12A  (via drill 0.5)
  Top 0.254: 77.22,49.34 MCP3208.12 76.61,48.71 76.34,48.71 75.77,48.14 75.77,40.45 76.69,39.52 v76.7,39.52 | R4.2 77.72,30.14 v77.72,37.33
  Bottom 0.254: v76.7,39.52 77.72,38.5 v77.72,37.34 v77.72,37.33
GPIO13  (via drill 0.48)
  Top 0.254: MCP3208.11 77.38,48.07 78.33,48.07 78.8,47.59 78.8,44.74 78.17,44.1 78.17,39.5 67.21,28.54 67.21,24.1 63.88,21.05 v63.82,21.12 61.98,20.92 ESP-12.15 | U$2.P$3 19.11,14.26 19.11,6.64 63.47,6.64 64.52,5.59 70.55,5.59 | AB8015.9 85.79,3.94 85.79,2.57 arc-90 84.37,1.08 70.56,1.08 70.55,5.59 | v64.23,19.05 68.48,19.18 69.91,17.75 69.91,14.38 70.55,13.75 70.55,5.59
  Bottom 0.254: v63.82,21.12 64.2,20.45 v64.23,19.05
GPIO14  (via drill 0.48, 0.5)
  Top 0.254: U$2.P$5 21.39,7.11 58.67,7.11 58.67,16.89 ESP-12.13 61.98,16.96 62,16.94 v64.85,17.83 | v67.81,22.68 67.8,22.7 65.28,20.13 v65.31,20.09 | MCP3208.13 77.22,50.61 76.1,50.61 75.31,49.82 75.31,37.43 66.05,28.17 66.05,24.92 66.04,24.91 v66.04,24.89 | v72.23,3.48 72.23,3.14 72.39,3.56 72.25,3.3 73.72,1.58 83.62,1.58 arc90 84.33,2.29 AB8015.7 arc90 AB8015.7
  Bottom 0.254: v64.85,17.83 v65.31,20.09 | v72.23,3.48 72.3,3.56 75.18,10.41 68.83,16.76 68.83,20.57 67.84,22.65 v67.81,22.68 66.12,24.82 v66.04,24.89
GPIO15  (via drill 0.5)
  Top 0.254: ESP-12.2 R3.1 47.88,20.89 v47.88,20.7 | v18.03,9.65 18.09,9.65 U$2.P$2
  Bottom 0.254: v47.88,20.7 45.35,20.7 41.25,16.6 41.25,9.65 v18.03,9.65
GPIO16
  Top 0.254: IO1.1 66.71,14.89 ESP-12.12
IND
  Top 1.016: TL2575HV.2 49.63,68.04 | 49.63,68.04 I1.P$1 | 49.63,68.04 49.63,65.1 D1.P$1
LOAD-NEG-A
  Top 0.406: 32.12,39.62 33.82,39.62 SHUNTMON-B.8 | C24.2 32.12,41.19 32.12,39.62 | J4.1 J4.2 J4.3 | 9.68,39.6 T2.1 21.87,39.62 32.12,39.62
  Top 2.54: J4.1 J4.3 9.68,39.6 | J4.2 7.11,42.06 U$1.P$2
LOAD-NEG-B
  Top 0.406: 32.51,53.59 33.82,53.59 SHUNTMON-A.8 | C23.2 32.51,54.88 32.51,53.59 | J1.3 9.68,53.57 T1.1 21.87,53.59 32.51,53.59
  Top 2.54: J1.1 J1.2 | J1.2 J1.3 | U$3.P$2 7.02,53.69 J1.2
N$1
  Top 0.254: MCP3208.5 68.12,49.33 59.69,40.89 SV1.1
N$2
  Top 0.406: 77.72,64.9 77.8,64.9 77.8,71.15
N$3
  Top 0.254: MCP3208.6 68.63,48.06 62.23,41.66 SV1.2
N$4
  Top 0.254: SHUNTMON-A.5 35.77,54.86 R13.1
N$5
  Top 0.254: MCP3208.7 69.14,46.79 64.77,42.42 SV1.3
N$6
  Top 0.254: SHUNTMON-B.5 35.81,40.81 R5.1
N$9
  Top 0.254: MCP3208.8 69.9,45.52 67.31,42.93 SV1.4
N$20  (via drill 0.48)
  Top 0.254: v75.56,22.67 79.79,23.08 80.07,24.1 B1.+$1 | v77.28,16.81 79.91,16.73 79.91,3.14 83.25,3.14 AB8015.5
  Bottom 0.254: v77.28,16.81 v75.56,22.67
N$22
  Top 0.254: Q1.4 83.32,7.32 AB8015.16
N$23
  Top 0.254: Q1.1 83.82,8.35 AB8015.15
N$30  (via drill 0.5)
  Top 0.254: v66.04,7.11 66.04,8.89 C21.2
  Bottom 0.254: FTDI1.1 60.2,7.11 v66.04,7.11
N$36  (via drill 0.5)
  Top 0.254: v39.97,10.94 R17.1
  Bottom 0.254: FTDI1.3 55.12,24.13 47.24,24.13 39.99,16.68 v39.97,10.94
PWR_IN
  Top 1.016: 44.27,66.33 TL2575HV.1 44.01,66.33 44.01,62.66 43.94,62.66 | PWR.2 9.46,62.66 21.93,62.66 | 43.94,62.66 42.29,62.66 41.9,62.27 | C16.1 41.9,62.27 | C17.1 43.97,62.63 43.94,62.66 | 21.93,62.66 C10.1 | 41.9,62.27 41.9,62.66 21.93,62.66
REF_A_INPUT
  Top 0.254: REF_SEL_A.2 37.93,44.79 35.05,41.91 | 35.05,41.91 35.05,40.07 SHUNTMON-B.6 | SHUNTMON-B.7 34.47,41.91 35.05,41.91
REF_B_INPUT
  Top 0.254: 36.2,57.28 35.05,56.13 | 35.05,56.13 35.05,54.04 SHUNTMON-A.6 | REF_SEL_B.2 36.2,57.28 | 36.2,57.28 | SHUNTMON-A.7 34.47,56.13 35.05,56.13
REF_INPUT  (via drill 0.5)
  Top 0.254: 43.69,50.04 v43.69,52.45 | 43.69,50.04 43.69,48.26 40.47,45.04 REF_SEL_A.1 | R10.1 R12.2 52.07,50.04 43.69,50.04
  Bottom 0.254: v43.69,52.45 43.69,55.63 40.13,59.18 39.01,59.18 REF_SEL_B.3
RESTESP
  Top 0.254: ESP-12.9 C21.1 64.43,10.83 R19.1
SOURCE-POS-A
  Top 0.254: R1.2 28.96,36.07
  Top 0.406: 32,36.07 28.96,36.07 28.96,36.1 T2.2 9.68,36.1 | 32,36.07 33.82,36.07 SHUNTMON-B.1 | C6.1 32,36.07 | J3.1 4.83,35.81 5.08,36.07 J3.2 J3.3
  Top 2.54: J3.1 J3.3 9.68,36.1 | J3.2 7.11,33.58 U$1.P$1
  Bottom 1.016: 22.86,36.07 21.87,36.07 T2.2 20.29,36.1 11.68,44.7 11.68,54.61 7.6,58.7 PWR.1
SOURCE-POS-B
  Top 0.254: R14.2 28.96,50.04
  Top 0.406: 32.26,50.04 28.96,50.04 28.96,50.07 T1.2 9.68,50.07 J2.3 J2.2 J2.1 | 32.26,50.04 33.69,50.04 33.82,49.91 SHUNTMON-A.1 | C25.1 32.26,50.04
  Top 2.54: J2.1 J2.3 | J2.2 7.11,47.63 U$3.P$1
  Bottom 1.016: PWR.3 12.68,57.17 19.81,50.04 21.82,50.04 T1.2
VSENSEA
  Top 0.254: R2.2 R1.1 | R2.2 37.69,31.08 38.48,31.88 43.72,31.88 57.69,45.85 62.45,45.85 67.21,50.61 71.82,50.61 MCP3208.4 | R2.2
VSENSEB
  Top 0.254: 28.96,44.96 R15.2 28.96,45.72 | R14.1 28.96,45.72 | MCP3208.2 69.03,53.14 68.58,53.59 42.93,53.59 41.91,52.58 41.91,48.01 40.64,46.74 34.04,46.74 33.02,45.72 28.96,45.72

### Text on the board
tPlace: VSENSE-B | VSENSE-A | MicroSD | TX/RX
bPlace: emonDC | wireless energy monitoring node | Technology that helps us live within ecological limits | Designed in North Wales UK by Megni | Lead free PCB - RoHS components | OpenEnergyMonitor.org | Node: | Designed in | North Wales | Made in UK | Open-Hardware | Format MicroSD / card to FAT32. / Place blank 'datalog.txt' / file there.
tNames: I1 | 470uF | 100uF | 16V | 80V | 330uH | D1 | A | USB_PWR | B | UNI | BI | B | LMP | UNI | BI | A | LMP | BOOT- / LOADER / MODE | FACTORY / RESET | GND / (0V)
tSilk: 5.0V | 4.7V | 4.7V | GND | 5V | Tx | Rx | RST | emonDCduo | Wireless Energy / Monitoring Node | v1.1 July 2017 by DB
_tsilk: Designed in | North Wales | Made in UK
_bsilk: SMT V0.6 rev3 | emonTx | wireless energy monitoring node | SMT V0.6 rev3 | emonTx | SMT V0.6 rev3 | emonTx | Technology that helps us live within ecological limits | wireless energy monitoring node | wireless energy monitoring node | Designed in North Wales UK by Glyn Hudson & Trystan Lea | Technology that helps us live within ecological limits | Technology that helps us live within ecological limits | Designed in North Wales UK by Glyn Hudson & Trystan Lea | 165mm ant | 433Mhz | Designed in North Wales UK by Glyn Hudson & Trystan Lea | 165mm ant | 165mm ant | 433Mhz | 433Mhz | 868Mhz | 82mm ant | 82mm ant | 82mm ant | 868Mhz | 868Mhz | 78mm ant | 915Mhz | 78mm ant | 915Mhz | 78mm ant | 915Mhz | 165mm ant | 433Mhz | 82mm ant | 868Mhz | 78mm ant | 915Mhz

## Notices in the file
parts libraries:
SparkFun-Connectors: Licensing: CC v3.0 Share-Alike You are welcome to use this library for commercial purposes.
SparkFun-Aesthetics: Licensing: Creative Commons ShareAlike 4.0 International - https://creativecommons.org/licenses/by-sa/4.0
